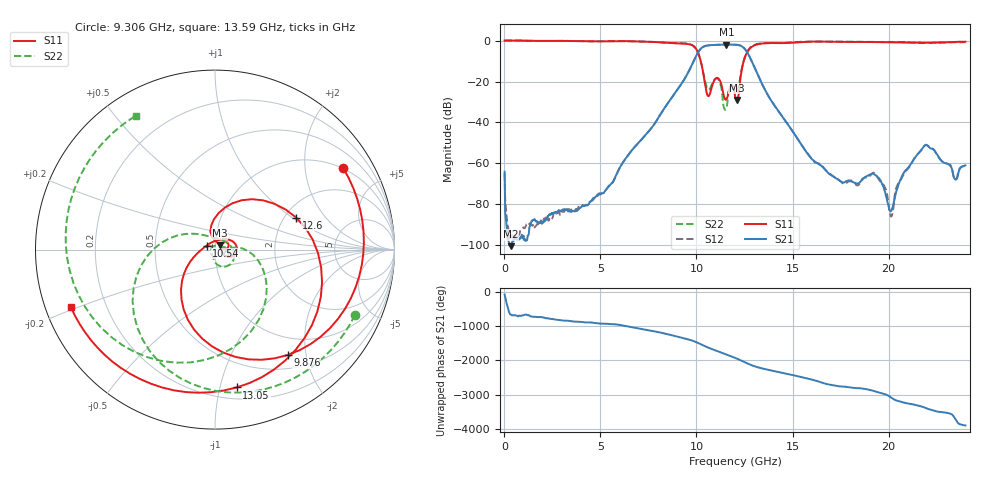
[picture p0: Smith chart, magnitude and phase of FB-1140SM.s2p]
! MARKI MICROWAVE INC.
! Email:  info@markimicrowave.com  Phone:  408-778-4200
! Model Number:  FB-1140SM  Date:  02/11
! Filename:		FB-1140SM.S2P  Version: 1.0
! Description:  2-port S-parameter data for Surface Mount Band Pass Filter FB-1140SM, measured in a connectorized fixture
! Frequency Range: 	10 MHz to 24 GHz
! Measurements:		S11, S21, S12, S22
# Hz S  dB  R 50
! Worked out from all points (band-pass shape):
!   801 points, 10 MHz to 24 GHz, reference 50 ohm
!   highest |S21| = -1.91 dB at 11.56 GHz (marker M1); lowest = -100.5 dB at 339.9 MHz (marker M2)
!   |S21| within 3 dB of the highest: 10.14 GHz to 12.58 GHz (2.443 GHz wide, 21.5 % of centre)
!   lowest |S11| = -29.0 dB at 12.09 GHz (marker M3), VSWR 1.07, Z = 52.6 + j2.6 ohm
!   |S11| at or under -10 dB: 10.22 GHz to 12.46 GHz (2.239 GHz wide, 19.7 % of centre)
!   |S22| runs from -33.8 to 0.1 dB; largest |S21 - S12| = 0.0019
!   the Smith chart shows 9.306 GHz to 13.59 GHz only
!   S11 on the Smith chart (normalised r, x): 9.306 GHz: 0.99, +3.16; 9.876 GHz: 0.70, -1.68; 10.54 GHz: 0.91, +0.04; 12.6 GHz: 2.30, +1.08; 13.05 GHz: 0.29, -1.13; 13.59 GHz: 0.08, -0.19
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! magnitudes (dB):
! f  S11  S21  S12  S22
! 10 MHz  0.0  -64.1  -64.9  0.1
! 339.9 MHz  0.1  -100.5  -96.3  0.1
! 4.028 GHz  -0.3  -80.9  -80.6  -0.3
! 5.558 GHz  -0.3  -70.0  -70.2  -0.2
! 8.017 GHz  -0.8  -37.7  -37.7  -0.8
! 9.306 GHz  -1.4  -19.8  -19.8  -1.3
! 9.876 GHz  -2.9  -9.6  -9.6  -2.8
! 10.54 GHz  -25.6  -2.4  -2.4  -22.9
! 11.11 GHz  -18.3  -2.1  -2.1  -18.7
! 11.56 GHz  -28.7  -1.9  -1.9  -33.1
! 12.01 GHz  -27.1  -2.0  -2.0  -24.4
! 12.09 GHz  -29.0  -2.1  -2.1  -25.0
! 12.6 GHz  -6.3  -5.2  -5.2  -6.1
! 13.05 GHz  -2.2  -13.9  -13.9  -1.9
! 13.59 GHz  -1.3  -24.5  -24.5  -1.2
! 16.02 GHz  -0.5  -58.0  -58.1  -0.5
! 17.67 GHz  -0.6  -69.3  -70.0  -0.5
! 19.26 GHz  -0.7  -65.4  -64.8  -0.7
! 20.01 GHz  -0.9  -81.5  -80.3  -0.6
! 21.9 GHz  -1.0  -51.1  -51.1  -1.1
! 23.49 GHz  -0.6  -67.9  -67.8  -0.8
! 24 GHz  -0.5  -61.0  -60.6  -0.8
